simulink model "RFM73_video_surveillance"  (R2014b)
settings: Solver=FixedStepDiscrete  StartTime=0.0  StopTime=5  FixedStep=1  RelTol=1e-3
libraries: simulink x1, embdlinuxlib x1

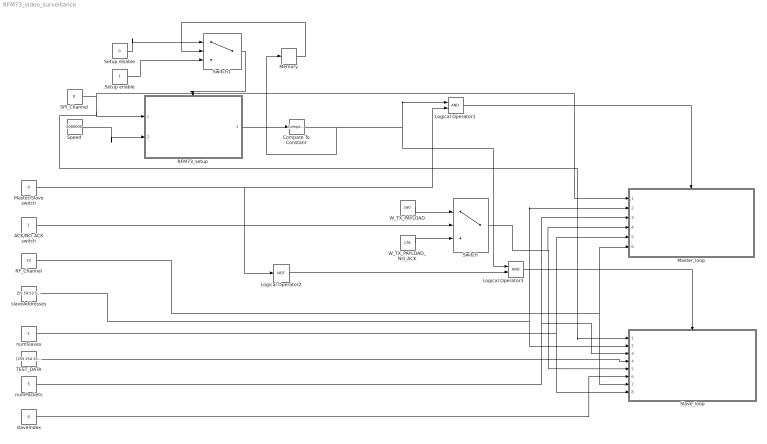
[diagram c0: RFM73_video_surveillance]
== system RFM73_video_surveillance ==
  ACK/NO_ACK switch : Constant
  Compare To Constant : simulink/Logic and Bit Operations/Compare To Constant  relop===  const=14  OutDataTypeStr=boolean
  Logical Operator1 : Logic  AllPortsSameDT=off  OutDataTypeStr=boolean
  Logical Operator2 : Logic  Operator=NOT  AllPortsSameDT=off  OutDataTypeStr=boolean
  Logical Operator3 : Logic  AllPortsSameDT=off  OutDataTypeStr=boolean
  Master/Slave switch : Constant  Value=0
  Master_loop : Subsystem  TreatAsAtomicUnit=on
  Memory : Memory
  RFM73_setup : Subsystem  TreatAsAtomicUnit=on
  RF_Channel : Constant  Value=23  OutDataTypeStr=uint8
  SPI_Channel : Constant  Value=0  OutDataTypeStr=uint8
  Setup disable : Constant  Value=0
  Setup enable : Constant
  Slave_loop : Subsystem  TreatAsAtomicUnit=on
  Speed : Constant  Value=2000000
  Switch : Switch  Criteria=u2 ~= 0
  Switch1 : Switch  Threshold=1
  TEST_DATA : Constant  Value=[255 254 253 252 251 250 255 254 253 252 251 250 255 254 253 252 251 250 255 254 253 252 251 250 255 254 253 252 251 250 255 254]  OutDataTypeStr=uint8
  W_TX_PAYLOAD : Constant  Value=160  OutDataTypeStr=uint8
  W_TX_PAYLOAD_NO_ACK : Constant  Value=176  OutDataTypeStr=uint8
  numPackets : Constant  Value=5  OutDataTypeStr=uint8
  numSlaves : Constant  OutDataTypeStr=uint8
  slaveAddresses : Constant  Value=[55 54 53 52 51 11 12 13 14 15]  OutDataTypeStr=uint8
  slaveIndex : Constant  Value=0  OutDataTypeStr=uint8
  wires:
  SPI_Channel/1 -> Master_loop/1(SPI), Slave_loop/1(SPI_Channel), RFM73_setup/1(SPI)
  Speed/1 -> RFM73_setup/2(Speed)
  Compare To Constant/1 -> Memory/1, Logical Operator1/1, Logical Operator3/1
  Master/Slave switch/1 -> Logical Operator2/1, Logical Operator1/2
  Logical Operator1/1 -> Master_loop/Enable
  ACK/NO_ACK switch/1 -> Switch/2
  W_TX_PAYLOAD/1 -> Switch/1
  W_TX_PAYLOAD_NO_ACK/1 -> Switch/3
  Switch/1 -> Master_loop/4(transmitMode), Slave_loop/5(transmitMode)
  TEST_DATA/1 -> Slave_loop/4(dataToSend)
  Logical Operator2/1 -> Logical Operator3/2
  Logical Operator3/1 -> Slave_loop/Enable
  Setup enable/1 -> Switch1/3
  RFM73_setup/1(StatusReg) -> Compare To Constant/1
  slaveAddresses/1 -> Slave_loop/2(Slave_address), Master_loop/2(slaveAddress)
  numPackets/1 -> Master_loop/3(nPackets), Slave_loop/3(nPackets)
  Memory/1 -> Switch1/2
  Setup disable/1 -> Switch1/1
  Switch1/1 -> RFM73_setup/Enable
  numSlaves/1 -> Slave_loop/8(nSlaves), Master_loop/5(nSlaves)
  slaveIndex/1 -> Slave_loop/6(slaveIndex)
  RF_Channel/1 -> Master_loop/6(RF_Channel), Slave_loop/7(RF_Channel)

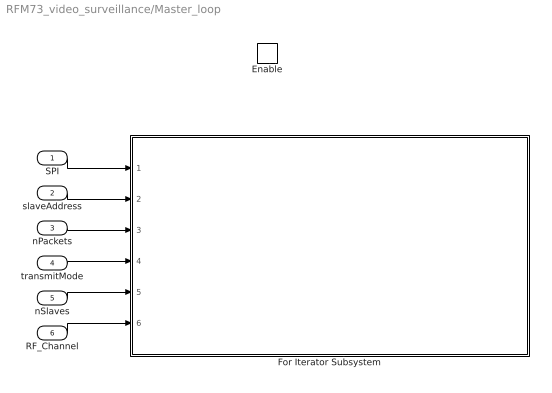
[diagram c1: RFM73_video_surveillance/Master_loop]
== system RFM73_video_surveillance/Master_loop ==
  SPI : Inport
  slaveAddress : Inport  Port=2
  nPackets : Inport  Port=3
  transmitMode : Inport  Port=4
  nSlaves : Inport  Port=5
  RF_Channel : Inport  Port=6
  Enable : EnablePort
  For Iterator Subsystem : Subsystem  TreatAsAtomicUnit=on
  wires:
  SPI/1 -> For Iterator Subsystem/1(SPI)
  slaveAddress/1 -> For Iterator Subsystem/2(slaveAddress)
  nPackets/1 -> For Iterator Subsystem/3(nPackets)
  transmitMode/1 -> For Iterator Subsystem/4(transmitMode)
  nSlaves/1 -> For Iterator Subsystem/5(nSlaves)
  RF_Channel/1 -> For Iterator Subsystem/6(RF_Channel)

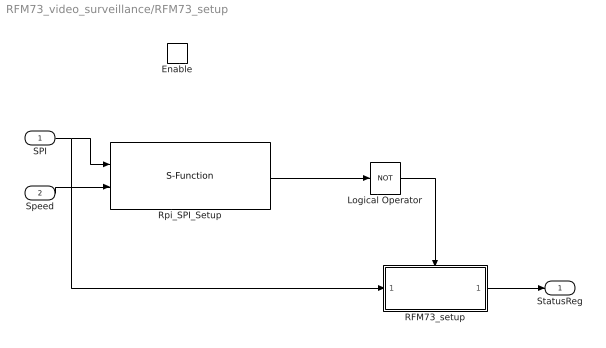
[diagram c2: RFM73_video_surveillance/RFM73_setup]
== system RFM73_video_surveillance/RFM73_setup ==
  SPI : Inport
  Speed : Inport  Port=2
  Enable : EnablePort
  Logical Operator : Logic  Operator=NOT  AllPortsSameDT=off  OutDataTypeStr=boolean
  RFM73_setup : Subsystem  TreatAsAtomicUnit=on
  Rpi_SPI_Setup : S-Function  InitFcn=try, set_param(gcb,'FunctionName','SPI_interface_setup'), end  FunctionName=SPI_interface_setup  SFunctionModules=SPI_interface_setup_wrapper  EnableBusSupport=off
  StatusReg : Outport
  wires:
  SPI/1 -> RFM73_setup/1(SPI), Rpi_SPI_Setup/1
  Speed/1 -> Rpi_SPI_Setup/2
  Rpi_SPI_Setup/1 -> Logical Operator/1
  Logical Operator/1 -> RFM73_setup/Enable
  RFM73_setup/1(Status_reg) -> StatusReg/1

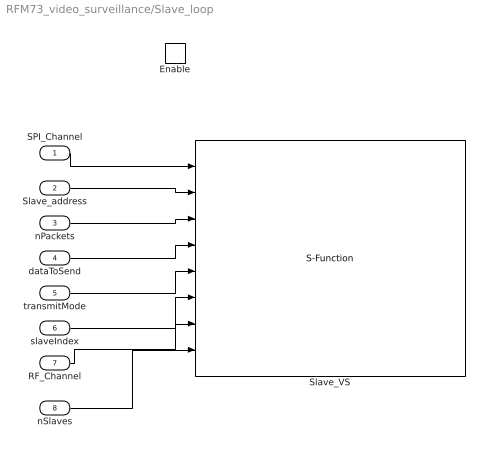
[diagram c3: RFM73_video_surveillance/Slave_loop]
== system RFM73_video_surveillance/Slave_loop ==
  SPI_Channel : Inport
  Slave_address : Inport  Port=2
  nPackets : Inport  Port=3
  dataToSend : Inport  Port=4
  transmitMode : Inport  Port=5
  slaveIndex : Inport  Port=6
  RF_Channel : Inport  Port=7
  nSlaves : Inport  Port=8
  Enable : EnablePort
  Slave_VS : S-Function  InitFcn=try, set_param(gcb,'FunctionName','RFM73_Slave_VS'), end  FunctionName=RFM73_Slave_VS  SFunctionModules=RFM73_Slave_VS_wrapper  EnableBusSupport=off
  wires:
  SPI_Channel/1 -> Slave_VS/1
  Slave_address/1 -> Slave_VS/2
  nPackets/1 -> Slave_VS/3
  dataToSend/1 -> Slave_VS/4
  transmitMode/1 -> Slave_VS/5
  slaveIndex/1 -> Slave_VS/6
  RF_Channel/1 -> Slave_VS/7
  nSlaves/1 -> Slave_VS/8

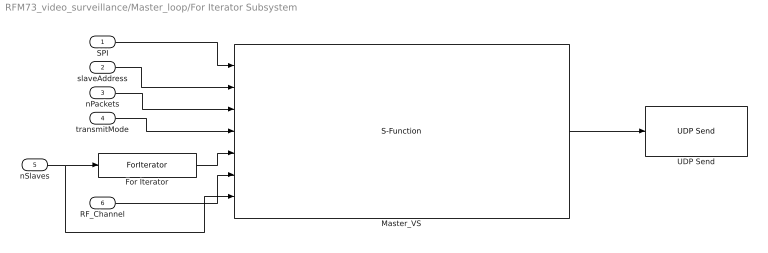
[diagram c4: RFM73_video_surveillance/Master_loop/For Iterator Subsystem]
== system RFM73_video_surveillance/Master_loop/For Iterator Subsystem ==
  SPI : Inport
  slaveAddress : Inport  Port=2
  nPackets : Inport  Port=3
  transmitMode : Inport  Port=4
  nSlaves : Inport  Port=5
  RF_Channel : Inport  Port=6
  For Iterator : ForIterator  IterationSource=external  IndexMode=Zero-based  IterationVariableDataType=int8
  Master_VS : S-Function  InitFcn=try, set_param(gcb,'FunctionName','RFM73_Master_VS'), end  FunctionName=RFM73_Master_VS  SFunctionModules=RFM73_Master_VS_wrapper  EnableBusSupport=off
  UDP Send : embdlinuxlib/UDP Send  remoteURL='169.254.0.1'  remotePort=25000  localURL='255.255.255.255'  localPortSource=Automatically determine  localPort=-1  sampletime=-1  blockPlatform=Raspberry Pi  separateLengthPort=0
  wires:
  SPI/1 -> Master_VS/1
  slaveAddress/1 -> Master_VS/2
  nPackets/1 -> Master_VS/3
  Master_VS/1 -> UDP Send/1
  transmitMode/1 -> Master_VS/4
  nSlaves/1 -> Master_VS/7, For Iterator/1
  For Iterator/1 -> Master_VS/5
  RF_Channel/1 -> Master_VS/6

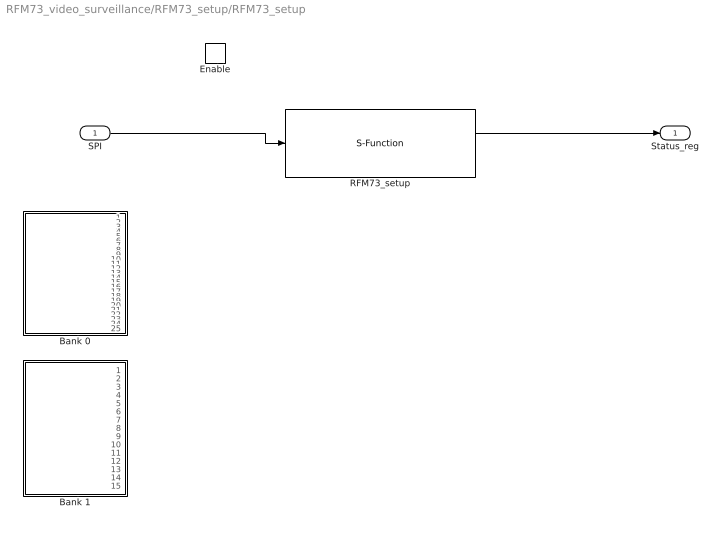
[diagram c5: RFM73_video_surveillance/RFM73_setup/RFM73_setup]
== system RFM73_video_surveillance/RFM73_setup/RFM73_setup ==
  SPI : Inport
  Enable : EnablePort
  Bank 0 : Subsystem
  Bank 1 : Subsystem
  RFM73_setup : S-Function  InitFcn=try, set_param(gcb,'FunctionName','setup'), end  FunctionName=setup  SFunctionModules=setup_wrapper  EnableBusSupport=off
  Status_reg : Outport
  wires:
  SPI/1 -> RFM73_setup/1
  RFM73_setup/1 -> Status_reg/1

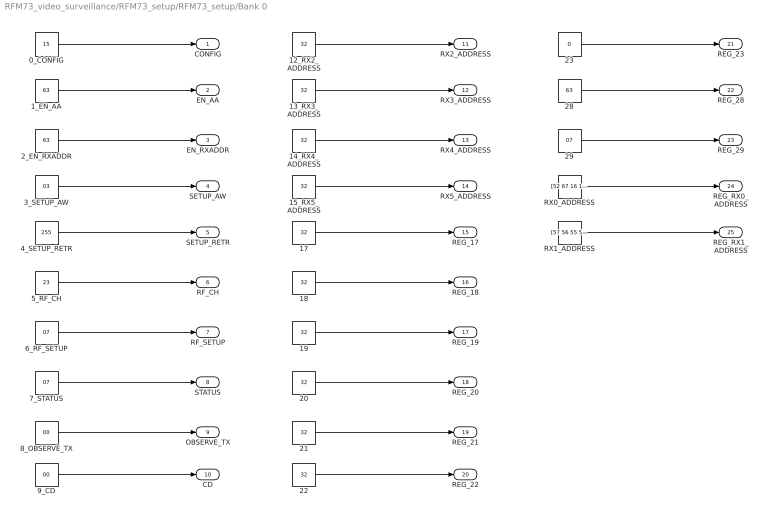
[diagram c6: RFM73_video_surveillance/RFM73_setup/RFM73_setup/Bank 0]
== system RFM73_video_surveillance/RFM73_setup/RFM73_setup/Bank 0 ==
  0_CONFIG : Constant  Value=15
  12_RX2_ADDRESS : Constant  Value=32
  13_RX3_ADDRESS : Constant  Value=32
  14_RX4_ADDRESS : Constant  Value=32
  15_RX5_ADDRESS : Constant  Value=32
  {17..22} (6 alike) : Constant  Value=32
  1_EN_AA : Constant  Value=63
  23 : Constant  Value=0
  28 : Constant  Value=63
  29 : Constant  Value=07
  2_EN_RXADDR : Constant  Value=63
  3_SETUP_AW : Constant  Value=03
  4_SETUP_RETR : Constant  Value=255
  5_RF_CH : Constant  Value=23
  6_RF_SETUP : Constant  Value=07
  7_STATUS : Constant  Value=07
  8_OBSERVE_TX : Constant  Value=00
  9_CD : Constant  Value=00
  RX0_ADDRESS : Constant  Value=[52 67 16 16 01]
  RX1_ADDRESS : Constant  Value=[57 56 55 54 178]
  CONFIG : Outport
  EN_AA : Outport  Port=2
  EN_RXADDR : Outport  Port=3
  SETUP_AW : Outport  Port=4
  SETUP_RETR : Outport  Port=5
  RF_CH : Outport  Port=6
  RF_SETUP : Outport  Port=7
  STATUS : Outport  Port=8
  OBSERVE_TX : Outport  Port=9
  CD : Outport  Port=10
  RX2_ADDRESS : Outport  Port=11
  RX3_ADDRESS : Outport  Port=12
  RX4_ADDRESS : Outport  Port=13
  RX5_ADDRESS : Outport  Port=14
  REG_17 : Outport  Port=15
  REG_18 : Outport  Port=16
  REG_19 : Outport  Port=17
  REG_20 : Outport  Port=18
  REG_21 : Outport  Port=19
  REG_22 : Outport  Port=20
  REG_23 : Outport  Port=21
  REG_28 : Outport  Port=22
  REG_29 : Outport  Port=23
  REG_RX0_ADDRESS : Outport  Port=24
  REG_RX1_ADDRESS : Outport  Port=25
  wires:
  0_CONFIG/1 -> CONFIG/1
  1_EN_AA/1 -> EN_AA/1
  2_EN_RXADDR/1 -> EN_RXADDR/1
  3_SETUP_AW/1 -> SETUP_AW/1
  4_SETUP_RETR/1 -> SETUP_RETR/1
  5_RF_CH/1 -> RF_CH/1
  6_RF_SETUP/1 -> RF_SETUP/1
  7_STATUS/1 -> STATUS/1
  8_OBSERVE_TX/1 -> OBSERVE_TX/1
  9_CD/1 -> CD/1
  12_RX2_ADDRESS/1 -> RX2_ADDRESS/1
  13_RX3_ADDRESS/1 -> RX3_ADDRESS/1
  14_RX4_ADDRESS/1 -> RX4_ADDRESS/1
  15_RX5_ADDRESS/1 -> RX5_ADDRESS/1
  18/1 -> REG_18/1
  19/1 -> REG_19/1
  17/1 -> REG_17/1
  23/1 -> REG_23/1
  28/1 -> REG_28/1
  29/1 -> REG_29/1
  20/1 -> REG_20/1
  21/1 -> REG_21/1
  22/1 -> REG_22/1
  RX0_ADDRESS/1 -> REG_RX0_ADDRESS/1
  RX1_ADDRESS/1 -> REG_RX1_ADDRESS/1

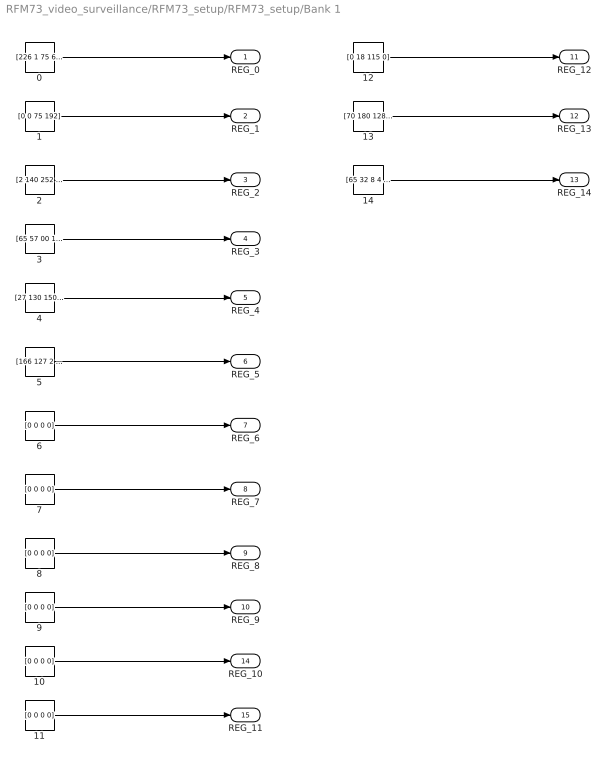
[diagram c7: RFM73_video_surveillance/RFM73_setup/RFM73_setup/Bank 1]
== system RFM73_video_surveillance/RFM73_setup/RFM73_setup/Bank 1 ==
  0 : Constant  Value=[226 1 75 64]
  1 : Constant  Value=[0 0 75 192]
  {6..11} (6 alike) : Constant  Value=[0 0 0 0]
  12 : Constant  Value=[0 18 115 0]
  13 : Constant  Value=[70 180 128 0]
  14 : Constant  Value=[65 32 8 4 129 32 207 247 254 255 255]
  2 : Constant  Value=[2 140 252 208]
  3 : Constant  Value=[65 57 00 153]
  4 : Constant  Value=[27 130 150 217]
  5 : Constant  Value=[166 127 2 36]
  REG_0 : Outport
  REG_1 : Outport  Port=2
  REG_2 : Outport  Port=3
  REG_3 : Outport  Port=4
  REG_4 : Outport  Port=5
  REG_5 : Outport  Port=6
  REG_6 : Outport  Port=7
  REG_7 : Outport  Port=8
  REG_8 : Outport  Port=9
  REG_9 : Outport  Port=10
  REG_12 : Outport  Port=11
  REG_13 : Outport  Port=12
  REG_14 : Outport  Port=13
  REG_10 : Outport  Port=14
  REG_11 : Outport  Port=15
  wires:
  0/1 -> REG_0/1
  1/1 -> REG_1/1
  2/1 -> REG_2/1
  3/1 -> REG_3/1
  4/1 -> REG_4/1
  5/1 -> REG_5/1
  6/1 -> REG_6/1
  7/1 -> REG_7/1
  8/1 -> REG_8/1
  9/1 -> REG_9/1
  12/1 -> REG_12/1
  13/1 -> REG_13/1
  14/1 -> REG_14/1
  10/1 -> REG_10/1
  11/1 -> REG_11/1
